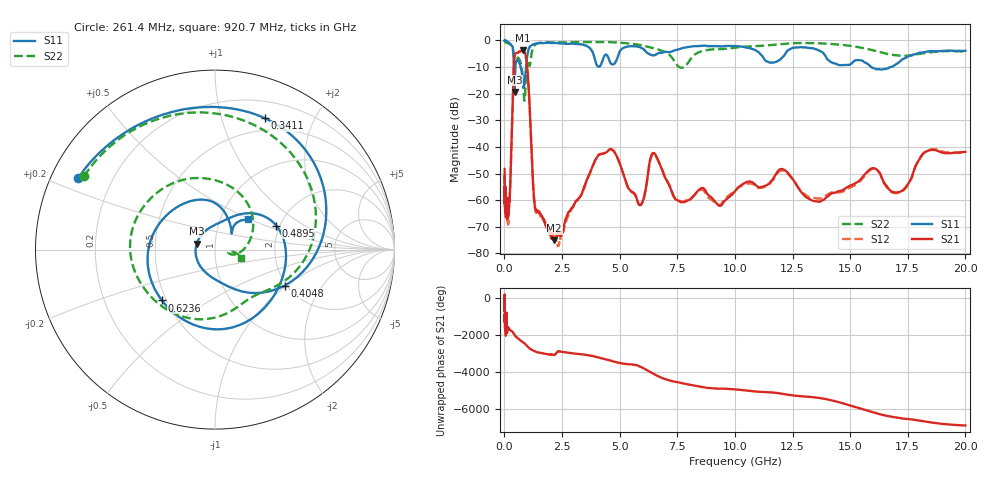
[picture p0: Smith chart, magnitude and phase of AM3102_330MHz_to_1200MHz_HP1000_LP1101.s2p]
! Date/Time: Tue, Sep 11, 2018 5:17 PM
! Network Analyzer: Agilent Technologies E8362B Rev: A.07.50.63
! Sweep from 0.010 to 20.000 GHz, 1601 Points, Sweep Type: LOG
! Power Supply: 4.949 V, 0.001 A
# Hz S DB R 50
!freq MagS11 AngS11 MagS21 AngS21 MagS12 AngS12 MagS22 AngS22
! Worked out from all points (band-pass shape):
!   1601 points, 10 MHz to 20 GHz, reference 50 ohm
!   highest |S21| = -3.78 dB at 794.6 MHz (marker M1); lowest = -75.1 dB at 2.165 GHz (marker M2)
!   |S21| within 3 dB of the highest: 427.7 MHz to 944.6 MHz (516.9 MHz wide, 75.3 % of centre)
!   lowest |S11| = -19.4 dB at 440.9 MHz (marker M3), VSWR 1.24, Z = 40.6 + j2.71 ohm
!   |S11| at or under -10 dB: 413.7 MHz to 476 MHz (62.3 MHz wide, 14 % of centre); 707.8 MHz to 941.8 MHz (234.1 MHz wide, 28.4 % of centre); 15.91 GHz to 16.77 GHz (858.9 MHz wide, 5.26 % of centre)
!   |S22| runs from -22.7 to -0.2 dB; largest |S21 - S12| = 0.01
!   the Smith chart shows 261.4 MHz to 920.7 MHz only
!   S11 on the Smith chart (normalised r, x): 261.4 MHz: 0.08, +0.24; 341.1 MHz: 0.37, +1.39; 404.8 MHz: 1.96, -0.97; 489.5 MHz: 1.92, +0.59; 623.6 MHz: 0.47, -0.32; 920.7 MHz: 1.35, +0.48
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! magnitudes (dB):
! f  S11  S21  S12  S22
! 10 MHz  0.0  -48.3  -53.6  -0.2
! 35.55 MHz  0.0  -62.0  -64.6  -0.5
! 126.4 MHz  -0.4  -63.5  -65.5  -1.0
! 261.4 MHz  -1.3  -52.6  -52.8  -1.6
! 341.1 MHz  -2.1  -28.8  -28.9  -2.6
! 404.8 MHz  -7.2  -10.5  -10.5  -6.0
! 440.9 MHz  -19.4  -5.7  -5.8  -9.4
! 447.2 MHz  -18.8  -5.4  -5.5  -9.5
! 489.5 MHz  -8.7  -4.9  -4.9  -8.0
! 623.6 MHz  -7.8  -4.3  -4.4  -6.8
! 794.6 MHz  -15.4  -3.8  -3.9  -13.7
! 920.7 MHz  -12.0  -5.6  -5.7  -16.3
! 1.302 GHz  -1.3  -60.6  -61.6  -1.9
! 1.59 GHz  -1.0  -65.6  -65.8  -0.9
! 2.165 GHz  -1.0  -75.1  -72.3  -0.7
! 4.5 GHz  -6.3  -41.4  -41.3  -0.6
! 5.652 GHz  -2.2  -57.6  -57.9  -1.4
! 6.518 GHz  -5.6  -42.5  -42.8  -3.0
! 7.625 GHz  -3.2  -60.6  -60.2  -10.2
! 12.03 GHz  -6.6  -48.3  -48.8  -1.4
! 13.61 GHz  -3.6  -60.6  -59.4  -1.1
! 20 GHz  -3.9  -41.9  -42.4  -4.2
